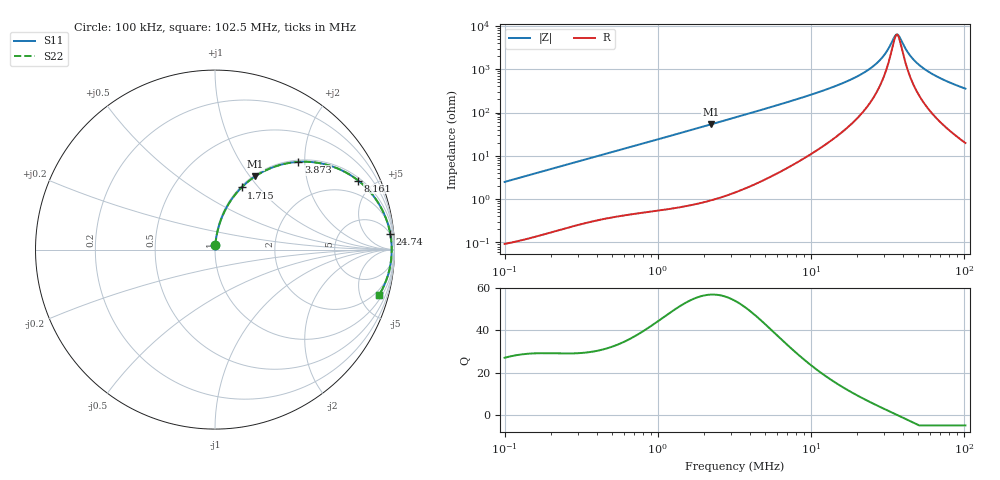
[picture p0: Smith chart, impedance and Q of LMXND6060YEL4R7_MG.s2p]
! LMXND6060YEL4R7_MG  S-PARAMETER MODEL  ( Standard Model )
! Model Generated by TAIYO YUDEN Corporation (http://www.ty-top.com)
! Version 1.0
! TAIYO YUDEN Control No. 20240226
! Copyright(c) 2024 TAIYO YUDEN CO.,LTD. All Rights Reserved.
! Product Description (link to TY-COMPAS)
! https://ds.yuden.co.jp/TYCOMPAS/or/detail?pn=LMXND6060YEL4R7NMG&u=M
! Products Name : Inductors
! Characteristics :
!  Inductance : 4.7 [uH] , SRF(min) : 25 [MHz] , DC Resistance(max) : 0.039 [Ohm]
!  Rated Current : Saturation  4400 [mA] , Temp Rise  3100 [mA] (40 [degC])
!  Case Size : 6.0 x 6.0 / 0.236 x 0.236 [mm/inch] , Thickness : 4.5 / 0.177 [mm/inch]
!  (Conditions: Temperature = 25 [degC] , DC Bias Current = 0 [A])
! External Node Assignments :
!  1  o---GGG---o  2
! GND o---------o GND
! Frequency Range : 0.1MHz  -  102.47202MHz  [ 402 STEP ]
# MHz S RI R 50
! Freq[MHz].  S11 Real  S11 Imag  S21 Real  S21 Imag  S12 Real  S12 Imag  S22 Real  S22 Imag
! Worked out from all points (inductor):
!   401 points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, 100 kHz to 102.5 MHz, reference 50 ohm
!   read as one part in series: L = 3.96 uH near 103.5 kHz
!   highest Q = 56.9 at 2.225 MHz (marker M1), where L = 3.8 uH
!   self-resonance near 36.23 MHz
!   S11 on the Smith chart (normalised r, x): 100 kHz: 1.00, +0.05; 1.715 MHz: 1.01, +0.82; 3.873 MHz: 1.04, +1.86; 8.161 MHz: 1.14, +4.08; 24.74 MHz: 5, +21; 102.5 MHz: 1.40, -7.10
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0.1  0.00154 0.0249  0.9985 -0.0249  0.9985 -0.0249  0.00154 0.0249
0.319357  0.00867 0.0772  0.9913 -0.0772  0.9913 -0.0772  0.00867 0.0772
1.019889  0.0607 0.2278  0.9393 -0.2278  0.9393 -0.2278  0.0607 0.2278
1.715332  0.148 0.3461  0.852 -0.3461  0.852 -0.3461  0.148 0.3461
2.224569  0.2241 0.4083  0.7759 -0.4083  0.7759 -0.4083  0.2241 0.4083
3.257086  0.3807 0.4763  0.6193 -0.4763  0.6193 -0.4763  0.3807 0.4763
3.873417  0.465 0.4889  0.535 -0.4889  0.535 -0.4889  0.465 0.4889
5.478032  0.6361 0.4689  0.3639 -0.4689  0.3639 -0.4689  0.6361 0.4689
8.160831  0.798 0.3846  0.202 -0.3846  0.202 -0.3846  0.798 0.3846
10.22302  0.8634 0.3224  0.1366 -0.3224  0.1366 -0.3224  0.8634 0.3224
17.1939  0.9508 0.1785  0.0492 -0.1785  0.0492 -0.1785  0.9508 0.1785
21.16862  0.968 0.1261  0.032 -0.1261  0.032 -0.1261  0.968 0.1261
24.74179  0.9764 0.0888  0.0236 -0.0888  0.0236 -0.0888  0.9764 0.0888
28.91811  0.9817 0.0529  0.0183 -0.0529  0.0183 -0.0529  0.9817 0.0529
32.64791  0.9839 0.0255  0.0161 -0.0255  0.0161 -0.0255  0.9839 0.0255
34.99141  0.9844 0.01  0.0156 -0.01  0.0156 -0.01  0.9844 0.01
36.85878  0.9846 -0.00156  0.0154 0.00156  0.0154 0.00156  0.9846 -0.00156
38.15874  0.9845 -0.00929  0.0155 0.00929  0.0155 0.00929  0.9845 -0.00929
44.59977  0.9826 -0.0443  0.0174 0.0443  0.0174 0.0443  0.9826 -0.0443
53.0393  0.9774 -0.084  0.0226 0.084  0.0226 0.084  0.9774 -0.084
69.98775  0.9608 -0.1511  0.0392 0.1511  0.0392 0.1511  0.9608 -0.1511
102.472  0.9146 -0.2529  0.0854 0.2529  0.0854 0.2529  0.9146 -0.2529
